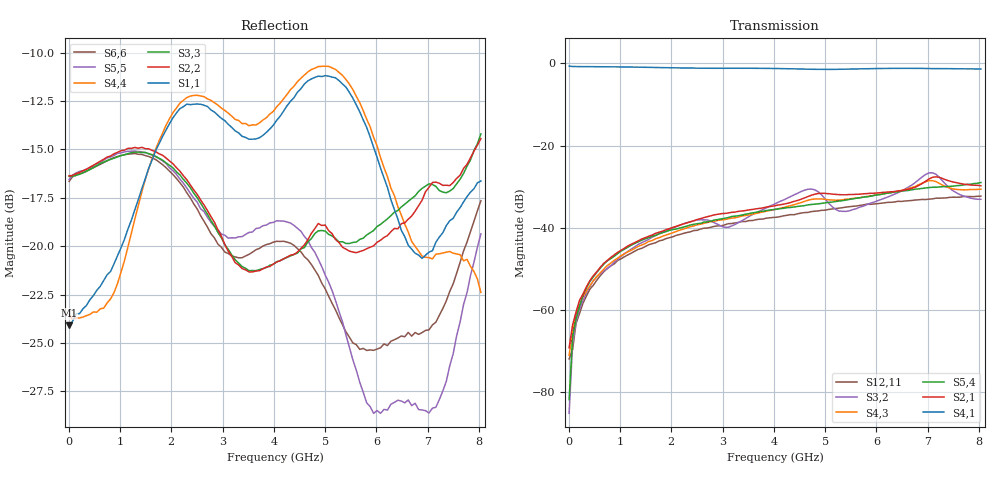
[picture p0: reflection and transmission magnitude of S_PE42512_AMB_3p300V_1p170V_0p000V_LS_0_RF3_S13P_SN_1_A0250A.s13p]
! Device ID: PE42512
! File Path: z:\PE42512\TE_GND_Post_Char_S-Param\All Parts\AMB\3p300\LS_0_RF3\PE42512_AMB_3p300V_1p170V_0p000V_LS_0_RF3_S13P_SN_1_A0250A.s13p
! Serial: 1
! Lot: A0250A
! Temp: AMB
! VDD: 3.300
! VSS: 0.000
! Control_Hi: 1.170
! Control_Lo: 0.000
! Logic State: LS_0_RF3
! Port 1:
! Port 2:
! Port 3:
! Port 4:
! Port 5:
! Port 6:
! Port 7:
! Port 8:
! Port 9:
! Port 10:
! Port 11:
! Port 12:
! Port 13:
! ThroughPath:1-4
! IDD: 0.0001068126
! ISS/IDD2: -2.62e-008
! IDMM3/IDD3: -2.028e-007
! Comment:
#  Hz  S  RI  R  50
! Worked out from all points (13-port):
!   120 points, 10 MHz to 8.037 GHz, reference 50 ohm
!   strongest paths, dB at 10 MHz, 2.034 GHz, 4.057 GHz, 6.08 GHz, 8.037 GHz:
!     S4,1: -0.7, -1.1, -1.2, -1.2, -1.4
!     S2,1: -69.2, -39.9, -34.6, -31.5, -29.8
!     S5,4: -81.9, -40.5, -35.5, -31.9, -29.0
!     S4,3: -71.1, -41.2, -35.5, -31.9, -30.6
!     S3,2: -85.2, -40.1, -34.0, -33.2, -33.1
!     S12,11: -72.0, -42.2, -37.5, -34.1, -32.3
!   lowest |S11| = -24.1 dB at 10 MHz (marker M1), VSWR 1.13, Z = 56.7 - j0.182 ohm
!   |S11| at or under -10 dB: start of sweep to end of sweep
